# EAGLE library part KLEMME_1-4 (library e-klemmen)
Klemme 4 Pol.
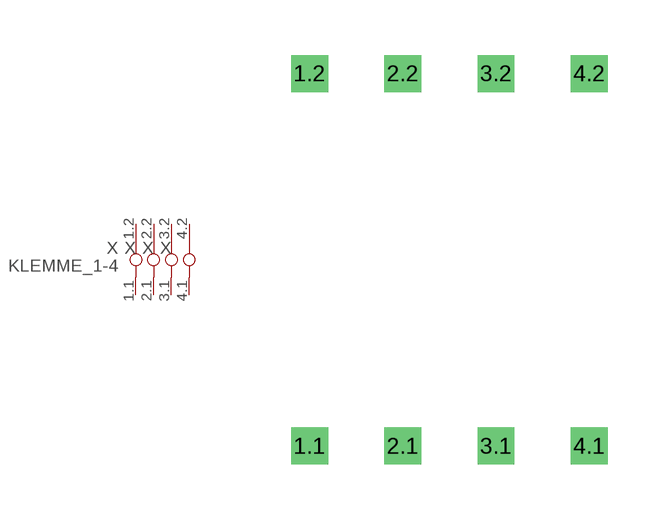
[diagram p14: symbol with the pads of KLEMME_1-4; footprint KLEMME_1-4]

Designator prefix X; gates 1=KLEMME_1-1 2=KLEMME_2 3=KLEMME_3 4=KLEMME_4

## KLEMME_1-4  [KLEMME_1-4]
1.1  1:1.1  pas
1.2  1:1.2  pas
2.1  2:2.1  pas
2.2  2:2.2  pas
3.1  3:3.1  pas
3.2  3:3.2  pas
4.1  4:4.1  pas
4.2  4:4.2  pas

## Footprint KLEMME_1-4 (pad centres in mm)
Dummy
drill 0.5 pad 1 square: 1.1 0,-12.7; 1.2 0,-2.54; 2.1 2.54,-12.7; 2.2 2.54,-2.54; 3.1 5.08,-12.7; 3.2 5.08,-2.54; 4.1 7.62,-12.7; 4.2 7.62,-2.54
